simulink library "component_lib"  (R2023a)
settings: Solver=VariableStepAuto  StartTime=0.0  StopTime=10.0  RelTol=1e-3
undefined symbols (not defined in the file or in its folder): component_lib, ECCV_r, KoblenzTrier, mm, par, param_TD04, R1234yf_ph, SigIdentifier, Systems, TH0023_WP120, Thermal, V_nom
libraries: base_lib x166, $bdroot x164, simulink x2, slpidlib x1
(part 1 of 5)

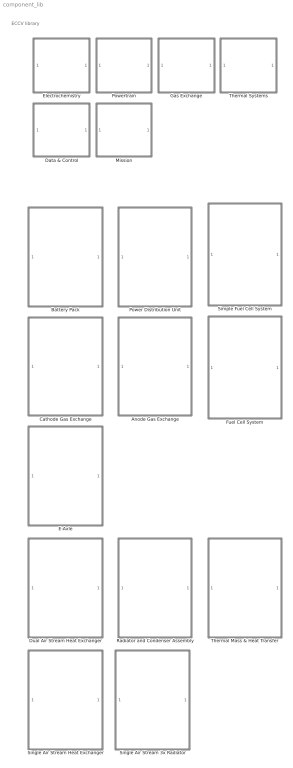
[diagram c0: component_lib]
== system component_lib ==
  note: ECCV library
  Anode Gas Exchange : Subsystem
  Battery Pack : Subsystem  mask{SOC_0=0.5, Nx=74, Ny=6*16}
      mask prompts: SOC_0 "Initial charge [-]:"; Nx "Cells in parallel  [-]:"; Ny "Cells in series [-]:"
      mask init:
      | % parameter struct
      | par = struct;
      | 
      | % Get user-defined parameters
      | par.Ny = eval(get_param(gcb, 'Ny'));
      | par.Nx = eval(get_param(gcb, 'Nx'));
  Cathode Gas Exchange : Subsystem
  Data & Control : Subsystem
  Dual Air Stream Heat Exchanger : Subsystem  mask{HtH=1.1, StS=0.95}
      mask prompts: HtH "Header to header [m]"; StS "Sideplate to sideplate [m]"
  E-Axle : Subsystem  mask{n=3, V_nom=700}
      mask prompts: n "Nr. of motors [-]"; V_nom "Nomnal voltage [V]:"
  Electrochemistry : Subsystem
  Fuel Cell System : Subsystem  mask{n_st=2, n=375}
      mask prompts: n_st "Stacks in series [#]:"; n "Cells per stack [#]:"
  Gas Exchange : Subsystem
  Mission : Subsystem
  Power Distribution Unit : Subsystem  mask{R_bf=1}
      mask prompts: R_bf "Burn-off resistance [Ohm]:"
  Powertrain : Subsystem
  Radiator and Condenser Assembly : Subsystem
  Simple Fuel Cell System : Subsystem  mask{n_st=2, n=375}
      mask prompts: n_st "Stacks in series [#]:"; n "Cells per stack [#]:"
  Single Air Stream 3x Radiator : Subsystem  mask{HtH=1.1, StS=0.95}
      mask prompts: HtH "Header to header [m]"; StS "Sideplate to sideplate [m]"
  Single Air Stream Heat Exchanger : Subsystem  mask{HtH=1.1, StS=0.95}
      mask prompts: HtH "Header to header [m]"; StS "Sideplate to sideplate [m]"
  Thermal Mass & Heat Transfer : Subsystem  mask{n=5, d=2e-3, L=50e-2, m=150, cp=420, T_0=273 + 20}
      mask prompts: n "Channels [-]:"; d "Hydraulic diameter [m]:"; L "Length [m]:"; m "Mass [kg]:"; cp "Heat capacity [J/kgK]:"; T_0 "Initial temperature [K]:"
  Thermal Systems : Subsystem

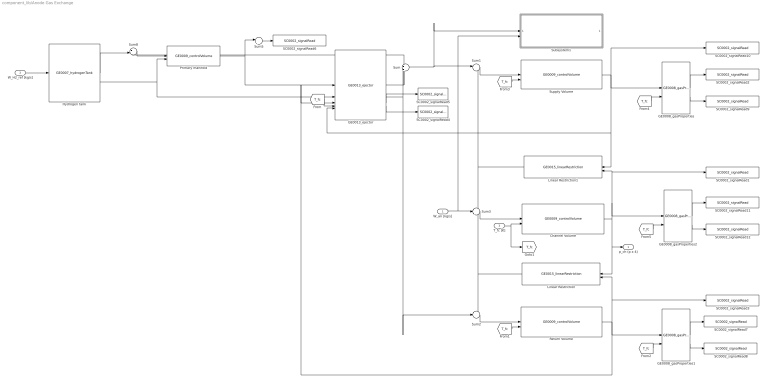
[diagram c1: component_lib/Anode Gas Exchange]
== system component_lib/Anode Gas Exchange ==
  W_an [kg/s] : Inport
  W_H2_ref [kg/s] : Inport  Port=2
  T_fc [K] : Inport  Port=3
  Channel Volume : $bdroot/Gas Exchange/GE0009_controlVolume  V=5e-3  p0=2.5e5  x0_H2=1  x0_O2=0  RH0=0.5
  GE0008_gasProperties : $bdroot/Gas Exchange/GE0008_gasProperties  SystemSampleTime=-1  VariantActivationTime=update diagram  Latency=0  AutoFrameSizeCalculation=off
  GE0008_gasProperties1 : $bdroot/Gas Exchange/GE0008_gasProperties  SystemSampleTime=-1  VariantActivationTime=update diagram  Latency=0  AutoFrameSizeCalculation=off
  GE0008_gasProperties2 : $bdroot/Gas Exchange/GE0008_gasProperties  SystemSampleTime=-1  VariantActivationTime=update diagram  Latency=0  AutoFrameSizeCalculation=off
  GE0013_ejector : $bdroot/Gas Exchange/GE0013_ejector  C_d=1  D_t=1.84e-3  Pi_lin=0.97  c_0=0.78406  c_1=-0.85801
  Hydrogen tank : $bdroot/Gas Exchange/GE0007_hydrogenTank  V=200e-3  T_tank=300  p_out=1.2e5  init_SOC=0.9  m0=5
  Linear Restriction : $bdroot/Gas Exchange/GE0015_linearRestriction  C_d=1e-5
  Linear Restriction1 : $bdroot/Gas Exchange/GE0015_linearRestriction  C_d=1e-5
  Primary manifold : $bdroot/Gas Exchange/GE0009_controlVolume  V=10e-3  p0=5e5  x0_H2=1  x0_O2=0  RH0=0.5
  Return Volume : $bdroot/Gas Exchange/GE0009_controlVolume  V=20e-3  p0=2.5e5  x0_H2=1  x0_O2=0  RH0=0.5
  SC0002_signalRead1 : $bdroot/Data & Control/SC0002_signalRead  SigName=anodeChannelPartialPressure
  SC0002_signalRead10 : $bdroot/Data & Control/SC0002_signalRead  SigName=anodeSupplyPartialPressure
  SC0002_signalRead11 : $bdroot/Data & Control/SC0002_signalRead  SigName=anodeChannelPressure
  SC0002_signalRead12 : $bdroot/Data & Control/SC0002_signalRead  SigName=anodeChannelHumidity
  SC0002_signalRead2 : $bdroot/Data & Control/SC0002_signalRead  SigName=anodeSupplyPressure
  SC0002_signalRead3 : $bdroot/Data & Control/SC0002_signalRead  SigName=anodeReturnPartialPressure
  SC0002_signalRead4 : $bdroot/Data & Control/SC0002_signalRead  SigName=entrainment
  SC0002_signalRead5 : $bdroot/Data & Control/SC0002_signalRead  SigName=recirculation
  SC0002_signalRead6 : $bdroot/Data & Control/SC0002_signalRead  SigName=anodePrimaryPressure
  SC0002_signalRead7 : $bdroot/Data & Control/SC0002_signalRead  SigName=anodeReturnPressure
  SC0002_signalRead8 : $bdroot/Data & Control/SC0002_signalRead  SigName=anodeReturnHumidity
  SC0002_signalRead9 : $bdroot/Data & Control/SC0002_signalRead  SigName=anodeSupplyHumidity
  Subsystem1 : Subsystem
  Sum : Sum  Inputs=+|+
  Sum1 : Sum  Inputs=|+-
  Sum2 : Sum  Inputs=+--
  Sum3 : Sum  Inputs=++-
  Sum5 : Sum  Inputs=1
  Sum8 : Sum  Inputs=-+|
  Supply Volume : $bdroot/Gas Exchange/GE0009_controlVolume  V=20e-3  p0=3e5  x0_H2=1  x0_O2=0  RH0=0.5
  p_ch (p x 4) : Outport
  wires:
  Sum1/1 -> Supply Volume/1
  GE0013_ejector/1 -> Sum/1, Sum8/1
  T_fc [K]/1 -> [T_fc], Channel Volume/2
  GE0013_ejector/4 -> SC0002_signalRead4/1
  GE0013_ejector/3 -> SC0002_signalRead5/1
  Hydrogen tank/2 -> Primary manifold/2, GE0013_ejector/2
  Sum8/1 -> Primary manifold/1
  Hydrogen tank/1 -> Sum8/2
  W_H2_ref [kg/s]/1 -> Hydrogen tank/1
  Sum5/1 -> SC0002_signalRead6/1
  Primary manifold/1 -> GE0013_ejector/1, Sum5/1
  GE0008_gasProperties/1 -> SC0002_signalRead2/1
  GE0013_ejector/2 -> Sum/2, Sum2/2
  Sum/1 -> Subsystem1/1(W_an), Sum1/1
  GE0008_gasProperties1/2 -> SC0002_signalRead8/1
  GE0008_gasProperties1/1 -> SC0002_signalRead7/1
  Linear Restriction/1 -> Sum3/3, Sum2/1
  Sum2/1 -> Return Volume/1
  Supply Volume/1 -> GE0013_ejector/5, Linear Restriction1/1, SC0002_signalRead10/1, GE0008_gasProperties/1
  Return Volume/1 -> SC0002_signalRead3/1, Linear Restriction/2, GE0013_ejector/3, GE0008_gasProperties1/1
  Sum3/1 -> Channel Volume/1
  Linear Restriction1/1 -> Sum1/2, Sum3/1
  W_an [kg/s]/1 -> Subsystem1/2(W_an_reacted), Sum3/2
  [T_fc] -> GE0013_ejector/4
  [T_fc] -> Return Volume/2
  [T_fc] -> GE0008_gasProperties1/2
  [T_fc] -> Supply Volume/2
  [T_fc] -> GE0008_gasProperties/2
  GE0008_gasProperties2/2 -> SC0002_signalRead12/1
  [T_fc] -> GE0008_gasProperties2/2
  Channel Volume/1 -> Linear Restriction/1, p_ch (p x 4)/1, GE0008_gasProperties2/1, SC0002_signalRead1/1, Linear Restriction1/2
  GE0008_gasProperties/2 -> SC0002_signalRead9/1
  GE0008_gasProperties2/1 -> SC0002_signalRead11/1

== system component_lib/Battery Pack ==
  I [A] : Inport
  T [K] : Inport  Port=2
  Battery current : $bdroot/Data & Control/SC0002_signalRead  SigName=batteryCurrent
  Cell current : $bdroot/Data & Control/SC0002_signalRead  SigName=batteryCellCurrent
  Cell voltage : $bdroot/Data & Control/SC0002_signalRead  SigName=batteryCellVoltage
  Constant1 : Constant  Value=Nx
  Constant2 : Constant  Value=Ny
  Constant4 : Constant  Value=Ny
  Constant5 : Constant  Value=Nx
  Divide : Product  Inputs=*/
  EL0001_panasonicNCR18650PF : $bdroot/Electrochemistry/EL0001_panasonicNCR18650PF  init_SOC=SOC_0
  Module voltage : $bdroot/Data & Control/SC0002_signalRead  SigName=batteryVoltage
  Module voltage1 : $bdroot/Data & Control/SC0002_signalRead  SigName=batteryPower
  Product1 : Product
  Product2 : Product  Inputs=3
  Product3 : Product
  SOC : $bdroot/Data & Control/SC0002_signalRead  SigName=stateOfCharge
  V [V] : Outport
  SOC [-] : Outport  Port=2
  Q_gen [J/s] : Outport  Port=3
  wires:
  Product1/1 -> Product3/2, Module voltage/1, V [V]/1
  EL0001_panasonicNCR18650PF/2 -> SOC/1, SOC [-]/1
  Constant2/1 -> Product1/1
  EL0001_panasonicNCR18650PF/1 -> Cell voltage/1, Product1/2
  Divide/1 -> EL0001_panasonicNCR18650PF/1, Cell current/1
  I [A]/1 -> Product3/1, Battery current/1, Divide/1
  Constant1/1 -> Divide/2
  T [K]/1 -> EL0001_panasonicNCR18650PF/2
  EL0001_panasonicNCR18650PF/3 -> Product2/1
  Constant5/1 -> Product2/3
  Constant4/1 -> Product2/2
  Product2/1 -> Q_gen [J/s]/1
  Product3/1 -> Module voltage1/1

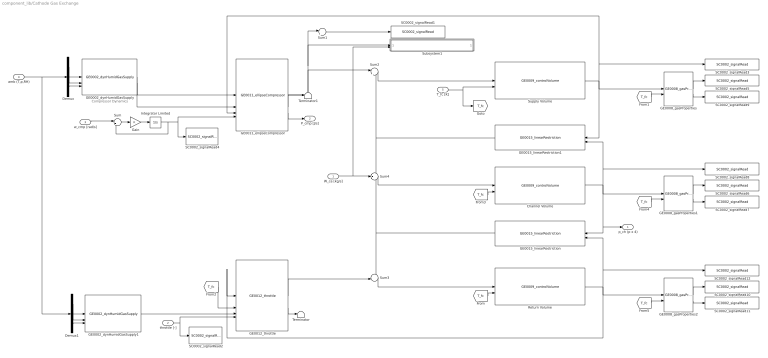
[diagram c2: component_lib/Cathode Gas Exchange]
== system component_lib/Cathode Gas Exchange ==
  note: Compressor Dynamics
  W_ca [kg/s] : Inport
  throttle [-] : Inport  Port=2
  w_cmp [rad/s] : Inport  Port=3
  amb (T,p,RH) : Inport  Port=4
  T_fc [K] : Inport  Port=5
  Channel Volume : $bdroot/Gas Exchange/GE0009_controlVolume  V=10e-3  p0=2.3e5  x0_H2=0  x0_O2=0.21  RH0=0.8
  Demux : Demux  Outputs=3
  Demux1 : Demux  Outputs=3
  GE0002_dynHumidGasSupply : $bdroot/Gas Exchange/GE0002_dynHumidGasSupply  x_H2_dry=0  x_O2_dry=0.21
  GE0002_dynHumidGasSupply1 : $bdroot/Gas Exchange/GE0002_dynHumidGasSupply  x_H2_dry=0  x_O2_dry=0.21
  GE0008_gasProperties : $bdroot/Gas Exchange/GE0008_gasProperties  SystemSampleTime=-1  VariantActivationTime=update diagram  Latency=0  AutoFrameSizeCalculation=off
  GE0008_gasProperties1 : $bdroot/Gas Exchange/GE0008_gasProperties  SystemSampleTime=-1  VariantActivationTime=update diagram  Latency=0  AutoFrameSizeCalculation=off
  GE0008_gasProperties2 : $bdroot/Gas Exchange/GE0008_gasProperties  SystemSampleTime=-1  VariantActivationTime=update diagram  Latency=0  AutoFrameSizeCalculation=off
  GE0011_ellipseCompressor : $bdroot/Gas Exchange/GE0011_ellipseCompressor  w0=15e3
  GE0012_throttle : $bdroot/Gas Exchange/GE0012_throttle  a0=1.3229e-05  a1=9.4736e-05  a2=0.0029  Pi_lin=0.97
  GE0015_linearRestriction : $bdroot/Gas Exchange/GE0015_linearRestriction  C_d=1e-5
  GE0015_linearRestriction1 : $bdroot/Gas Exchange/GE0015_linearRestriction  C_d=1e-5
  Gain : Gain
  Integrator Limited : Integrator  InitialCondition=1e4  LimitOutput=on  UpperSaturationLimit=2e4  LowerSaturationLimit=3e3
  Return Volume : $bdroot/Gas Exchange/GE0009_controlVolume  V=40e-3  p0=2e5  x0_H2=0  x0_O2=0.21  RH0=0.8
  SC0002_signalRead1 : $bdroot/Data & Control/SC0002_signalRead  SigName=compressorFlow
  SC0002_signalRead10 : $bdroot/Data & Control/SC0002_signalRead  SigName=cathodeReturnPressure
  SC0002_signalRead11 : $bdroot/Data & Control/SC0002_signalRead  SigName=cathodeReturnHumidity
  SC0002_signalRead12 : $bdroot/Data & Control/SC0002_signalRead  SigName=cathodeReturnPartialPressure
  SC0002_signalRead2 : $bdroot/Data & Control/SC0002_signalRead  SigName=throttlePosition
  SC0002_signalRead3 : $bdroot/Data & Control/SC0002_signalRead  SigName=cathodeSupplyPartialPressure
  SC0002_signalRead4 : $bdroot/Data & Control/SC0002_signalRead  SigName=compressorSpeed
  SC0002_signalRead5 : $bdroot/Data & Control/SC0002_signalRead  SigName=cathodeSupplyPressure
  SC0002_signalRead6 : $bdroot/Data & Control/SC0002_signalRead  SigName=cathodeChannelPressure
  SC0002_signalRead7 : $bdroot/Data & Control/SC0002_signalRead  SigName=cathodeChannelHumidity
  SC0002_signalRead8 : $bdroot/Data & Control/SC0002_signalRead  SigName=cathodeChannelPartialPressure
  SC0002_signalRead9 : $bdroot/Data & Control/SC0002_signalRead  SigName=cathodeSupplyHumidity
  Subsystem1 : Subsystem
  Sum : Sum  Inputs=|+-
  Sum1 : Sum  Inputs=1
  Sum2 : Sum  Inputs=|+-
  Sum3 : Sum  Inputs=+-|
  Sum4 : Sum  Inputs=++-
  Supply Volume : $bdroot/Gas Exchange/GE0009_controlVolume  V=40e-3  p0=2.5e5  x0_H2=0  x0_O2=0.21  RH0=0.8
  Terminator : Terminator
  Terminator1 : Terminator
  p_ch (p x 4) : Outport
  P_cmp [J/s] : Outport  Port=2
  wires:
  Sum1/1 -> SC0002_signalRead1/1
  Gain/1 -> Integrator Limited/1
  Integrator Limited/1 -> SC0002_signalRead4/1, GE0011_ellipseCompressor/4, Sum/2
  Sum/1 -> Gain/1
  w_cmp [rad/s]/1 -> Sum/1
  GE0002_dynHumidGasSupply/1 -> GE0011_ellipseCompressor/1
  GE0002_dynHumidGasSupply1/1 -> GE0012_throttle/3
  GE0002_dynHumidGasSupply/2 -> GE0011_ellipseCompressor/2
  GE0011_ellipseCompressor/1 -> Sum2/1, Sum1/1, Subsystem1/1(W_ca)
  throttle [-]/1 -> SC0002_signalRead2/1, GE0012_throttle/4
  Demux/1 -> GE0002_dynHumidGasSupply/1
  Demux/2 -> GE0002_dynHumidGasSupply/2
  Demux/3 -> GE0002_dynHumidGasSupply/3
  Demux1/1 -> GE0002_dynHumidGasSupply1/1
  Demux1/2 -> GE0002_dynHumidGasSupply1/2
  Demux1/3 -> GE0002_dynHumidGasSupply1/3
  amb (T,p,RH)/1 -> Demux/1, Demux1/1
  GE0008_gasProperties/1 -> SC0002_signalRead5/1
  Supply Volume/1 -> GE0015_linearRestriction1/1, GE0008_gasProperties/1, GE0011_ellipseCompressor/3, SC0002_signalRead3/1
  GE0008_gasProperties/2 -> SC0002_signalRead9/1
  Sum2/1 -> Supply Volume/1
  GE0011_ellipseCompressor/3 -> P_cmp [J/s]/1
  GE0015_linearRestriction/1 -> Sum4/3, Sum3/1
  T_fc [K]/1 -> [T_fc], Supply Volume/2
  Sum3/1 -> Return Volume/1
  GE0012_throttle/1 -> Sum3/2
  GE0012_throttle/2 -> Terminator/1
  GE0011_ellipseCompressor/2 -> Terminator1/1
  [T_fc] -> Return Volume/2
  [T_fc] -> GE0008_gasProperties/2
  [T_fc] -> GE0012_throttle/2
  Channel Volume/1 -> p_ch (p x 4)/1, GE0015_linearRestriction/1, GE0008_gasProperties1/1, GE0015_linearRestriction1/2, SC0002_signalRead8/1
  W_ca [kg/s]/1 -> Sum4/2, Subsystem1/2(W_ca_reacted)
  GE0015_linearRestriction1/1 -> Sum4/1, Sum2/2
  Sum4/1 -> Channel Volume/1
  [T_fc] -> Channel Volume/2
  [T_fc] -> GE0008_gasProperties1/2
  GE0008_gasProperties1/1 -> SC0002_signalRead6/1
  GE0008_gasProperties1/2 -> SC0002_signalRead7/1
  GE0008_gasProperties2/1 -> SC0002_signalRead10/1
  GE0008_gasProperties2/2 -> SC0002_signalRead11/1
  [T_fc] -> GE0008_gasProperties2/2
  Return Volume/1 -> GE0008_gasProperties2/1, GE0012_throttle/1, GE0015_linearRestriction/2, SC0002_signalRead12/1

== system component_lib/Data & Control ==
  DC0007_cathodeFlowControl : Subsystem  mask{lambda_O2_ref=2, n_cell=455}
      mask prompts: lambda_O2_ref "Oxygen stoich. reference [-]:"; n_cell "Nr. of cells [-]:"
  SC0002_signalRead : Subsystem  mask{SigName=SigIdentifier}
      mask prompts: SigName "Signal identifier:"
      mask init:
      | % set name of input port
      | blockNames = Simulink.findBlocks(gcb);
      | set(blockNames(1), 'Name', SigName);
      | 
      | % log input port
      | ph = get_param([gcb, '/', SigName], 'PortHandles');
      | set_param(ph.Outport(1), 'DataLogging', 'on')
      | 
      | % set signal name in goto tag
      | set_param([gcb, '/', 'Goto'], 'GotoTag', SigName)
  SC0003_signalWrite : Subsystem  mask{SigName=SigIdentifier}
      mask prompts: SigName "Signal identifier:"
      mask init:
      | % set signal name in goto tag
      | set_param([gcb, '/', 'From'], 'GotoTag', SigName)

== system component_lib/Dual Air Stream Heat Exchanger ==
  AMB: (T,p,RH) : Inport
  v [m/s] : Inport  Port=2
  Q_cds [J/s] : Inport  Port=3
  rel_fan_speed [-] : Inport  Port=4
  CL: (T1,p1,W1) : Inport  Port=5
  Demux : Demux  Outputs=3
  Mux : Mux  Inputs=3
  Radiator core - behind CDS : $bdroot/Thermal Systems/TH0002_radiatorCore  HtH=0.35  StS=0.95  radmodel=52 mm
  Radiator core - exposed : $bdroot/Thermal Systems/TH0002_radiatorCore  HtH=1.1-0.35  StS=0.95  radmodel=52 mm
  TH0003_coolantTank : $bdroot/Thermal Systems/TH0003_coolantTank  StS=0.95  D_con=0.055  T_0=286  radmodel=52 mm
  TH0003_coolantTank1 : $bdroot/Thermal Systems/TH0003_coolantTank  StS=0.95  D_con=0.055  T_0=286  radmodel=52 mm
  TH0004_radiatorPlugFlow : $bdroot/Thermal Systems/TH0004_radiatorPlugFlow  HtH=1.1  StS=0.95  T_0=286  radmodel=52 mm
  TH0005_flowSplit : $bdroot/Thermal Systems/TH0005_flowSplit  SystemSampleTime=-1  VariantActivationTime=update diagram  Latency=0  AutoFrameSizeCalculation=off
  TH0006_flowConfluence : $bdroot/Thermal Systems/TH0006_flowConfluence  gain=0.01
  TH0007_airRestriction : $bdroot/Thermal Systems/TH0007_airRestriction  A=0.8  zeta=0.3
  TH0007_airRestriction1 : $bdroot/Thermal Systems/TH0007_airRestriction  A=1  zeta=2.5
  TH0008_condenser : $bdroot/Thermal Systems/TH0008_condenser  HtH=0.85  StS=0.35  cdsmodel=18.8 mm
  TH0009_intake : $bdroot/Thermal Systems/TH0009_intake  zeta=0.9
  TH0010_fan : $bdroot/Thermal Systems/TH0010_fan  n_fan=4
  TH0011_outletFlowBalance : $bdroot/Thermal Systems/TH0011_outletFlowBalance  gain=0.05
  P_fan [J/s] : Outport
  CL: (T2,p2,W2) : Outport  Port=2
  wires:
  Demux/2 -> Mux/2, [p_amb]
  Demux/1 -> Mux/1
  AMB: (T,p,RH)/1 -> Demux/1
  TH0003_coolantTank1/1 -> CL: (T2,p2,W2)/1
  TH0010_fan/2 -> P_fan [J/s]/1
  rel_fan_speed [-]/1 -> TH0010_fan/2
  TH0005_flowSplit/1 -> TH0008_condenser/1
  v [m/s]/1 -> TH0009_intake/2
  TH0007_airRestriction/1 -> TH0005_flowSplit/1
  TH0004_radiatorPlugFlow/1 -> TH0003_coolantTank1/1
  TH0007_airRestriction1/1 -> TH0011_outletFlowBalance/1
  TH0003_coolantTank/1 -> Radiator core - behind CDS/2
  Q_cds [J/s]/1 -> TH0008_condenser/2
  CL: (T1,p1,W1)/1 -> TH0003_coolantTank/1
  TH0006_flowConfluence/2 -> TH0005_flowSplit/2
  TH0006_flowConfluence/1 -> TH0010_fan/1
  Mux/1 -> TH0009_intake/1
  TH0005_flowSplit/2 -> [air_22]
  TH0009_intake/1 -> TH0007_airRestriction/1
  TH0008_condenser/1 -> Radiator core - behind CDS/1
  Radiator core - behind CDS/2 -> TH0006_flowConfluence/1
  Radiator core - exposed/2 -> TH0006_flowConfluence/2
  Radiator core - behind CDS/3 -> Radiator core - exposed/2
  [p_amb] -> TH0011_outletFlowBalance/2
  [air_22] -> Radiator core - exposed/1
  TH0010_fan/1 -> TH0007_airRestriction1/1
  Radiator core - exposed/3 -> TH0004_radiatorPlugFlow/1
  TH0011_outletFlowBalance/1 -> [W_in]
  [W_in] -> Mux/3

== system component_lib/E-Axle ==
  note: Input as % of max. torque at current speed
  Tq_sig [-] : Inport
  gear [-] : Inport  Port=2
  V [V] : Inport  Port=3
  w_w [rad/s] : Inport  Port=4
  Constant1 : Constant  Value=V_nom
  Constant3 : Constant
  Current sensor : $bdroot/Data & Control/SC0002_signalRead  SigName=motorCurrent
  Divide : Product  Inputs=**/
  Divide1 : Product  Inputs=**
  Gain : Gain  Gain=n
  Gain1 : Gain  Gain=n
  Gain2 : Gain  Gain=n
  Gain3 : Gain  Gain=-1
  Max torque : $bdroot/Data & Control/SC0002_signalRead  SigName=maxMotorTorque
  Min torque : $bdroot/Data & Control/SC0002_signalRead  SigName=minMotorTorque
  PT0002_simpleMotor : $bdroot/Powertrain/PT0002_simpleMotor  T_s=0.1
  PT0003_gearBox : $bdroot/Powertrain/PT0003_gearBox  fd_ratio=2  gear_ratios=[5 3.8 2.3 1.15]  eta_gb=0.98
  Saturation2 : Saturate  UpperLimit=1  LowerLimit=-1
  Saturation3 : Saturate  UpperLimit=476  LowerLimit=0
  Saturation4 : Saturate  UpperLimit=V_nom  LowerLimit=0
  Speed sensor : $bdroot/Data & Control/SC0002_signalRead  SigName=motorSpeed
  Torque sensor : $bdroot/Data & Control/SC0002_signalRead  SigName=motorTorque
  speed-Torque map1 : Lookup_n-D  NumberOfTableDimensions=1  BreakpointsForDimension1=|  Table=|  ExtrapMethod=Clip  UseLastTableValue=on  InternalRulePriority=Speed  RndMeth=Simplest
      | [25.2590673575129
      | 34.9740932642487
      | 43.3937823834197
      | 51.1658031088083
      | 55.6994818652850
      | 64.1191709844560
      | 65.4145077720207
      | 67.3575129533679
      | 68.0051813471503
      | 69.9481865284974
      | 71.2435233160622
      | 73.1865284974093
      | 75.7772020725389
      | 76.4248704663213
      | 78.3678756476684
      | 81.6062176165803
      | 82.9015544041451
      | 86.1398963730570
      | 88.0829015544041
      | 90.0259067357513
      | 94.5595854922280
      | 97.1502590673575
      | 100.388601036269
      | 103.6269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
      | [1991.26637554585
      | 1997.08879184862
      | 1994.17758369723
      | 1994.17758369723
      | 1994.17758369723
      | 1991.26637554585
      | 1944.68704512373
      | 1921.39737991266
      | 1854.43959243086
      | 1816.59388646288
      | 1787.48180494905
      | 1700.14556040757
      | 1671.03347889374
      | 1621.54294032023
      | 1548.76273653566
      | 1513.82823871907
      | 1438.13682678311
      | 1391.55749636099
      | 1339.15574963610
      | 1280.93158660844
      | 1225.61863173217
      | 1176.12809315866
      | 1129.54876273654
      | 1085.880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
  Tq_axle [Nm] : Outport
  I_em [A] : Outport  Port=2
  Q_gen [J/s] : Outport  Port=3
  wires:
  Gain2/1 -> Tq_axle [Nm]/1
  PT0003_gearBox/1 -> Gain2/1
  PT0002_simpleMotor/3 -> Gain/1
  Gain1/1 -> Current sensor/1, I_em [A]/1
  PT0002_simpleMotor/1 -> PT0003_gearBox/1, Torque sensor/1
  Constant3/1 -> PT0003_gearBox/4
  gear [-]/1 -> PT0003_gearBox/3
  PT0003_gearBox/2 -> Divide/1, PT0002_simpleMotor/3, Speed sensor/1
  w_w [rad/s]/1 -> PT0003_gearBox/2
  PT0002_simpleMotor/2 -> Gain1/1
  Gain/1 -> Q_gen [J/s]/1
  Gain3/1 -> Min torque/1
  V [V]/1 -> PT0002_simpleMotor/2, Saturation4/1
  speed-Torque map1/1 -> Divide1/2, Gain3/1, Max torque/1
  Saturation2/1 -> Divide1/1
  Saturation4/1 -> Divide/3
  Saturation3/1 -> speed-Torque map1/1
  Divide1/1 -> PT0002_simpleMotor/1
  Tq_sig [-]/1 -> Saturation2/1
  Constant1/1 -> Divide/2
  Divide/1 -> Saturation3/1

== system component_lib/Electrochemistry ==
  EL0001_panasonicNCR18650PF : Subsystem  mask{init_SOC=0.2380}
      mask prompts: init_SOC "Initial SOC [-]:"
      mask init:
      | % parameter struct
      | par = struct;
      | 
      | % Get user-defined parameters
      | par.init_SOC   = init_SOC;
  EL0004_buckCCM : Subsystem  mask{R=1e-3, C=1, L=1e-6, V_init=400}
      mask prompts: R "Resistance [Ohm]:"; C "Capacity [F]:"; L "Inductance [H]:"; V_init "Voltage initial condition [V]:"
  EL0005_boostCCM : Subsystem  mask{C=1, L=1, eta=0.9, V_init=420}
      mask prompts: C "Capacity [F]:"; L "Inductance [H]:"; eta "Efficiency [-]:"; V_init "Voltage initial condition [V]:"
  EL0006_busDC : Subsystem  mask{R=1e-3, C=1, L=912e-9, V_init=420}
      mask prompts: R "Resistance [Ohm]:"; C "Capacitance [F]:"; L "Inductance [H]:"; V_init "Voltage initial condition [V]:"
  EL0007_pukrushpan2004 : Subsystem  mask{U_0=1, j_0=1e-3, alpha=0.25, ASR=1e-1, A_fc=300}
      mask prompts: U_0 "Open circuit voltage [V]:"; j_0 "Exchange current density [A/cm2]:"; alpha "Act. bar. symmetry [-]:"; ASR "Area specific resistance [ohm*cm2]:"; A_fc "Membrane area [cm2]:"
      mask init:
      | % parameter struct
      | par = struct;
      | 
      | % Get user-defined parameters
      | par.j_0   = j_0;
      | par.alpha = alpha;
      | par.ASR   = ASR;
      | par.U_0   = U_0;
      | par.A_fc  = A_fc;
      | 
      | % membrane thickness
      | par.t_m    = 0.01275;
      | 
      | % Molar mass - [kg/mol]
      | par.M_j  = [0.002;
      |             0.032;
      |             0.018;
      |             0.028];    
      | 
      | % Specific heat - [J/kg*K]        
      | par.cp_j = [14.43e3;
      |             0.928e3;
      |             1.996e3;
      |             1.041e3];  
      | 
      | % Universal gas constant - [J/(mol*K)]   
      | par.R  = 8.314;         
      | 
      | % Specific gas constant [J/kg*K]
      | par.R_j = par.R ./ par.M_j;
  EL0008_dcdcConverter : Subsystem  mask{eta_up=0.99, eta_down=0.99}
      mask prompts: eta_up "Efficiency up [-]"; eta_down "Efficiency down [-]"
      mask init:
      | par = struct;
      | par.eta_up = eta_up;
      | par.eta_down = eta_down;
  EL0010_superCapacitor : Subsystem  mask{C=1, V_bus0=700}
      mask prompts: C "Capacity [F]:"; V_bus0 "Initial voltage [V]:"

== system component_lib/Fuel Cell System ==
  I [A] : Inport
  throttle [-] : Inport  Port=2
  w_cmp [rad/s] : Inport  Port=3
  W_H2_ref [kg/s] : Inport  Port=4
  amb (T,p,RH) : Inport  Port=5
  T [K] : Inport  Port=6
  Anode Gas Exchange : $bdroot/Anode Gas Exchange  SystemSampleTime=-1  VariantActivationTime=update diagram  Latency=0  AutoFrameSizeCalculation=off
  Cathode Gas Exchange : $bdroot/Cathode Gas Exchange  SystemSampleTime=-1  VariantActivationTime=update diagram  Latency=0  AutoFrameSizeCalculation=off
  Constant4 : Constant  Value=n
  EL0007_pukrushpan2004 : $bdroot/Electrochemistry/EL0007_pukrushpan2004  U_0=1  j_0=1e-3  alpha=0.25  ASR=1e-1  A_fc=420
  F0010_vaporSaturationPressure.m : base_lib/F0010_gasFlow/F0010_vaporSaturationPressure.m  SystemSampleTime=-1  VariantActivationTime=update diagram  Latency=0  AutoFrameSizeCalculation=off
  Gain{,1..3} (4 alike) : Gain  Gain=n_st
  Gain4 : Gain  Gain=1/420
  Product{1..5} (5 alike) : Product
  SC0002_signalRead1 : $bdroot/Data & Control/SC0002_signalRead  SigName=fuelCellVoltage
  SC0002_signalRead2 : $bdroot/Data & Control/SC0002_signalRead  SigName=fuelCellCurrent
  SC0002_signalRead3 : $bdroot/Data & Control/SC0002_signalRead  SigName=membraneWaterContent
  SC0002_signalRead4 : $bdroot/Data & Control/SC0002_signalRead  SigName=fuelCellPower
  SC0002_signalRead5 : $bdroot/Data & Control/SC0002_signalRead  SigName=vaporSaturationPressure
  SC0002_signalRead6 : $bdroot/Data & Control/SC0002_signalRead  SigName=singleCellVoltage
  SC0002_signalRead7 : $bdroot/Data & Control/SC0002_signalRead  SigName=compressorPower
  SC0002_signalRead8 : $bdroot/Data & Control/SC0002_signalRead  SigName=currentDensity
  Subsystem1 : Subsystem
  V [V] : Outport
  Q_gen [J/s] : Outport  Port=2
  P_cmp [J/s] : Outport  Port=3
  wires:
  Product1/1 -> Gain1/1
  EL0007_pukrushpan2004/1 -> Product1/1, SC0002_signalRead6/1
  Product2/1 -> [W_an], Gain/1
  Product5/1 -> [W_ca]
  Constant4/1 -> Product1/2, Product2/2, Product5/2, Product3/2
  I [A]/1 -> EL0007_pukrushpan2004/1, SC0002_signalRead2/1, Product4/1, Gain4/1
  EL0007_pukrushpan2004/3 -> Product5/1
  EL0007_pukrushpan2004/2 -> Product2/1
  EL0007_pukrushpan2004/5 -> Product3/1
  Product4/1 -> SC0002_signalRead4/1
  EL0007_pukrushpan2004/4 -> SC0002_signalRead3/1
  T [K]/1 -> F0010_vaporSaturationPressure.m/1, Anode Gas Exchange/3, Cathode Gas Exchange/5, EL0007_pukrushpan2004/4, EL0007_pukrushpan2004/5, EL0007_pukrushpan2004/6
  Cathode Gas Exchange/2 -> Gain3/1
  amb (T,p,RH)/1 -> Cathode Gas Exchange/4
  F0010_vaporSaturationPressure.m/1 -> SC0002_signalRead5/1
  Cathode Gas Exchange/1 -> EL0007_pukrushpan2004/3
  [W_ca] -> Cathode Gas Exchange/1
  Gain3/1 -> SC0002_signalRead7/1, P_cmp [J/s]/1
  Gain/1 -> Subsystem1/1(In1)
  Gain1/1 -> V [V]/1, SC0002_signalRead1/1, Product4/2
  Product3/1 -> Gain2/1
  Gain2/1 -> Q_gen [J/s]/1
  throttle [-]/1 -> Cathode Gas Exchange/2
  w_cmp [rad/s]/1 -> Cathode Gas Exchange/3
  Anode Gas Exchange/1 -> EL0007_pukrushpan2004/2
  [W_an] -> Anode Gas Exchange/1
  Gain4/1 -> SC0002_signalRead8/1
  W_H2_ref [kg/s]/1 -> Anode Gas Exchange/2

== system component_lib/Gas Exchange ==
  GE0001_humidGasSupply : Subsystem  mask{p_tot=1.01e5, x_H2=0, x_O2=0.21, RH=0, T=300}
      mask prompts: p_tot "Pressure [Pa]:"; x_H2 "Mole fraction dry H2 [-]:"; x_O2 "Mole fraction dry O2 [-]:"; RH "Relative humidity [-]:"; T "Temperature [K]:"
      mask init:
      | % parameter struct
      | par = struct;
      | 
      | par.p_tot = p_tot;
      | par.x_H2  = x_H2;
      | par.x_O2  = x_O2;
      | par.RH    = RH;
      | par.T     = T;
      | 
      | % par.p_tot = eval(get_param(gcb, 'p_tot'));
      | % par.x_H2  = eval(get_param(gcb, 'x_H2'));
      | % par.x_O2  = eval(get_param(gcb, 'x_O2'));
      | % par.RH    = eval(get_param(gcb, 'RH'));
      | % par.T     = eval(get_param(gcb, 'T'));
      | 
      | 
      | 
      | % Fixed parameters
      | par.R     = 8.314;  % [J/(mol*K)] - universal gas constant
      | par.M_N2  = 0.028;  % [kg/mol] - nitrogen molecular weight
      | par.M_H2O = 0.018;  % [kg/mol] - water
  GE0002_dynHumidGasSupply : Subsystem  mask{x_H2_dry=0, x_O2_dry=0.21}
      mask prompts: x_H2_dry "Mole-fraction dry hydrogen [-]:"; x_O2_dry "Mole-fraction dry oxygen [-]:"
      mask init:
      | % parameter struct
      | par = struct;
      | 
      | % Fixed parameters
      | par.R     = 8.314; % [J/(mol*K)] - universal gas constant
      | par.M_N2  = 0.028; % [kg/mol] - nitrogen molecular weight
      | par.M_H2O = 0.018; % [kg/mol] - water
  GE0007_hydrogenTank : Subsystem  mask{V=200e-3, T_tank=300, p_out=1.2e5, init_SOC=0.9, m0=5}
      mask prompts: V "Volume [m3]:"; T_tank "Tank temperature [K]:"; p_out "Outlet pressure [Pa]"; init_SOC "Initial charge [-]"; m0 "Total capacity [kg]:"
      mask init:
      | % parameter struct
      | par = struct;
      | 
      | % Get user-specified parameters
      | % par.V        = eval(get_param(gcb, 'V'));
      | % par.T_tank   = eval(get_param(gcb, 'T_tank'));
      | % par.p_out    = eval(get_param(gcb, 'p_out'));
      | % par.init_SOC = eval(get_param(gcb, 'init_SOC'));
      | % par.m0       = eval(get_param(gcb, 'm0'));
      | 
      | par.V        = V;
      | par.T_tank   = T_tank;
      | par.p_out    = p_out;
      | par.init_SOC = init_SOC;
      | par.m0       = m0;
      | 
      | 
      | % Standard state values
      | par.T0 = 298.15;  % [K]     - standard state temperature
      | par.h0 = 7.9260e3; % [J/mol] - standard state enthalpy
      | 
      | % Molar mass - [kg/mol]
      | par.M_j  = [0.002;
      |             0.032;
      |             0.018;
      |             0.028];    
      | 
      | % Specific heat - [J/kg*K]        
      | par.cp_j = [14.43e3;
      |             0.928e3;
      |             1.996e3;
      |             1.041e3];  
      | 
      | % Universal gas constant - [J/(mol*K)]   
      | par.R  = 8.314;         
      | 
      | % Specific gas constant [J/kg*K]
      | par.R_j = par.R ./ par.M_j;
  GE0008_gasProperties : Subsystem
  GE0009_controlVolume : Subsystem  mask{V=1.5833e-05, p0=1.01e5, x0_H2=0, x0_O2=0.21, RH0=0}
      mask prompts: V "Volume [m3]:"; p0 "Pressure [Pa]:"; x0_H2 "Mole fraction dry H2 [-]:"; x0_O2 "Mole fraction dry O2 [-]:"; RH0 "Relative humidity [-]:"
      mask init:
      | % parameter struct
      | par = struct;
      | 
      | % Get user-specified parameters
      | % par.V   = eval(get_param(gcb, 'V'));
      | par.V = V;
      | 
      | % initial conditions
      | par.p0    = p0;
      | par.x0_H2 = x0_H2;
      | par.x0_O2 = x0_O2;
      | par.RH0   = RH0;
      | 
      | % Molar mass - [kg/mol]
      | par.M_j  = [0.002;
      |             0.032;
      |             0.018;
      |             0.028];    
      | 
      | % Specific heat - [J/kg*K]        
      | par.cp_j = [14.43e3;
      |             0.928e3;
      |             1.996e3;
      |             1.041e3];  
      | 
      | % Universal gas constant - [J/(mol*K)]   
      | par.R  = 8.314;         
      | 
      | % Specific gas constant [J/kg*K]
      | par.R_j = par.R ./ par.M_j;
  GE0010_compressibleRestriction : Subsystem  mask{C_d=1, D_t=1.84e-3, Pi_lin=0.97}
      mask prompts: C_d "Discharge coefficient [-]:"; D_t "Throat diameter [m]:"; Pi_lin "Lin. region  [-]"
      mask init:
      | % Check side
      | par = struct;
      | 
      | % parameters
      | par.C_d     = C_d;
      | par.Pi_lin  = Pi_lin;
      | par.D_t     = D_t;
      | 
      | % Molar mass - [kg/mol]
      | par.M_j  = [0.002;
      |             0.032;
      |             0.018;
      |             0.028];    
      | 
      | % Specific heat - [J/kg*K]        
      | par.cp_j = [14.43e3;
      |             0.928e3;
      |             1.996e3;
      |             1.041e3];  
      | 
      | % Universal gas constant - [J/(mol*K)]   
      | par.R  = 8.314;         
      | 
      | % Specific gas constant [J/kg*K]
      | par.R_j = par.R ./ par.M_j;
  GE0011_ellipseCompressor : Subsystem  mask{compressor_parameters=param_TD04.mat, w0=3e3}
      mask prompts: compressor_parameters "Parameter set:"; w0 "Initial speed [rad/s]:"
      mask init:
      | % parameter struct
      | % par = struct;
      | 
      | 
      | 
      | % find compressor models
      | compressorMaps = dir(fullfile('models/F0011_ellipseCompressor','*.mat'));
      | compressorMaps = {compressorMaps.name};
      | 
      | % update popup_list
      | msk = Simulink.Mask.get(gcb);
      | msk.Parameters(1).TypeOptions = compressorMaps;
      | 
      | % set profile
      | % try
      |     load(msk.Parameters(1).Value);
      | % end
      | 
      | % Get user-specified parameters
      | % par.w0   = eval(get_param(gcb, 'w0'));
      | par.w0   = w0;
      | 
      | 
      | % % Compressor parameters
      | % par.C_Wch       = [0.791459084209095;0.278369840595707;2.56393896117876;1.42688664691882];
      | % par.C_PIch      = [0.0903657853262553;0.467638667413134;4.35616456423884]; 
      | % par.C_Wzs       = [0.851951915665070;2.98625689994966];
      | % par.C_PIzs      = [1.24697676678299;2.08506798865712];
      | % par.C_cur       = [2.08068646432419;4.30416619749832;5.84893356036723];
      | % par.Gamma_PIcs  = [0.500000000000000];
      | % par.C_s         = [1.47023010236244];
      | % par.C_b         = [1.806586538255675;-0.642454577867690];
      | % par.C_a         = [0.863755184943499;0.033339263835893;24.999999984802365];
      | % par.C_loss      = 0.009455201151738;
      | % par.T_ref       =  298;
      | % par.p_ref       = 100000;
      | % par.Nc_max_map  = 1.860592187500000e+05;
      | % par.Wc_max_map  = 0.252151000000000;
      | % par.PI_max_map  = 2.766539113153419;
      | % par.Delta_h_max = 1.738661132271557e+05;
      | % par.gamma_air   = 1.397693997445722;
      | % par.rho1        = 1.169072149521521;
      | % par.D_2         = 0.056300000000000;
      | % par.Cp_air      = 1.008800956523303e+03;
      | % par.alpha_kPiW0 = 1.645763320284325;
      | % par.J_c         = 1.730000000000000e-05;
      | % par.c_fric      = 1e-6;
      | 
      | 
      | % Molar mass - [kg/mol]
      | par.M_j  = [0.002;
      |             0.032;
      |             0.018;
      |             0.028];    
      | 
      | % Specific heat - [J/kg*K]        
      | par.cp_j = [14.43e3;
      |             0.928e3;
      |             1.996e3;
      |             1.041e3];  
      | 
      | % Universal gas constant - [J/(mol*K)]   
      | par.R  = 8.314;         
      | 
      | % Specific gas constant [J/kg*K]
      | par.R_j = par.R ./ par.M_j;
  GE0012_throttle : Subsystem  mask{a0=1.3229e-05, a1=9.4736e-05, a2=0.0029, Pi_lin=0.97}
      mask prompts: Pi_lin "Lin. region  [-]"
      mask init:
      | % Check side
      | par = struct;
      | 
      | % parameters
      | par.Pi_lin  = Pi_lin;
      | 
      | par.C_d = 1;
      | par.a0 = a0;
      | par.a1 = a1;
      | par.a2 = a2;
      | 
      | % Molar mass - [kg/mol]
      | par.M_j  = [0.002;
      |             0.032;
      |             0.018;
      |             0.028];    
      | 
      | % Specific heat - [J/kg*K]        
      | par.cp_j = [14.43e3;
      |             0.928e3;
      |             1.996e3;
      |             1.041e3];  
      | 
      | % Universal gas constant - [J/(mol*K)]   
      | par.R  = 8.314;         
      | 
      | % Specific gas constant [J/kg*K]
      | par.R_j = par.R ./ par.M_j;
  GE0013_ejector : Subsystem  mask{C_d=1, D_t=1.84e-3, Pi_lin=0.97, c_0=0.78406, c_1=-0.85801}
      mask prompts: C_d "Discharge coefficient [-]:"; D_t "Nozzle throat diameter [m]:"; Pi_lin "Linear region [-]:"; c_0 "c0"; c_1 "c1"
      mask init:
      | % parameter struct
      | par = struct;
      | 
      | % Get user-specified parameters
      | % par.C_d    = eval(get_param(gcb, 'C_d'));
      | % par.D_t    = eval(get_param(gcb, 'D_t'));
      | % par.Pi_lin = eval(get_param(gcb, 'Pi_lin'));
      | % par.c_0     = eval(get_param(gcb, 'c_0'));
      | % par.c_1     = eval(get_param(gcb, 'c_1'));
      | 
      | par.C_d    = C_d;
      | par.D_t    = D_t;
      | par.Pi_lin = Pi_lin;
      | par.c_0    = c_0;
      | par.c_1    = c_1;
      |  
      | % Molar mass - [kg/mol]
      | par.M_j  = [0.002;
      |             0.032;
      |             0.018;
      |             0.028];    
      | 
      | % Specific heat - [J/kg*K]        
      | par.cp_j = [14.43e3;
      |             0.928e3;
      |             1.996e3;
      |             1.041e3];  
      | 
      | % Universal gas constant - [J/(mol*K)]   
      | par.R  = 8.314;         
      | 
      | % Specific gas constant [J/kg*K]
      | par.R_j = par.R ./ par.M_j;
  GE0014_flowValve : Subsystem  mask{C_d=1, D_t=1.84e-3, Pi_lin=0.97}
      mask prompts: C_d "Discharge coefficient [-]:"; D_t "Throat diameter [m]:"; Pi_lin "Lin. region  [-]"
      mask init:
      | % Check side
      | par = struct;
      | 
      | % parameters
      | par.C_d     = C_d;
      | par.Pi_lin  = Pi_lin;
      | par.D_t     = D_t;
      | 
      | % Molar mass - [kg/mol]
      | par.M_j  = [0.002;
      |             0.032;
      |             0.018;
      |             0.028];    
      | 
      | % Specific heat - [J/kg*K]        
      | par.cp_j = [14.43e3;
      |             0.928e3;
      |             1.996e3;
      |             1.041e3];  
      | 
      | % Universal gas constant - [J/(mol*K)]   
      | par.R  = 8.314;         
      | 
      | % Specific gas constant [J/kg*K]
      | par.R_j = par.R ./ par.M_j;
  GE0015_linearRestriction : Subsystem  mask{C_d=4.7083e-08}
      mask prompts: C_d "Discharge coefficient [-]:"
      mask init:
      | % Check side
      | par = struct;
      | 
      | % parameters
      | % par.C_d     = eval(get_param(gcb, 'C_d'));
      | % par.tan_par = eval(get_param(gcb, 'tan_par'));
      | 
      | par.C_d     = C_d;
      | 
      | % Molar mass - [kg/mol]
      | par.M_j  = [0.002;
      |             0.032;
      |             0.018;
      |             0.028];    
      | 
      | % Specific heat - [J/kg*K]        
      | par.cp_j = [14.43e3;
      |             0.928e3;
      |             1.996e3;
      |             1.041e3];  
      | 
      | % Universal gas constant - [J/(mol*K)]   
      | par.R  = 8.314;         
      | 
      | % Specific gas constant [J/kg*K]
      | par.R_j = par.R ./ par.M_j;
  GE0016_simpleCompressor : Subsystem  mask{eta=0.7}
      mask prompts: eta "Efficiency [-]:"
  GE0017_humidifier : Subsystem  mask{T_s=30, gain=1}
      mask prompts: T_s "Time constant [s]:"; gain "Gain [RH -> Flow]:"
      mask init:
      | % parameter struct
      | par = struct;
      | 
      | 
      | % Molar mass - [kg/mol]
      | par.M_j  = [0.002;
      |             0.032;
      |             0.018;
      |             0.028];    
      | 
      | % Specific heat - [J/kg*K]        
      | par.cp_j = [14.43e3;
      |             0.928e3;
      |             1.996e3;
      |             1.041e3];  
      | 
      | % Universal gas constant - [J/(mol*K)]   
      | par.R  = 8.314;         
      | 
      | % Specific gas constant [J/kg*K]
      | par.R_j = par.R ./ par.M_j;
  GE0018_condenser : Subsystem  mask{T_s=1, gain=1}
      mask prompts: T_s "Time constant [s]:"; gain "Gain [RH -> Flow]:"
      mask init:
      | % parameter struct
      | par = struct;
      | 
      | 
      | % Molar mass - [kg/mol]
      | par.M_j  = [0.002;
      |             0.032;
      |             0.018;
      |             0.028];    
      | 
      | % Specific heat - [J/kg*K]        
      | par.cp_j = [14.43e3;
      |             0.928e3;
      |             1.996e3;
      |             1.041e3];  
      | 
      | % Universal gas constant - [J/(mol*K)]   
      | par.R  = 8.314;         
      | 
      | % Specific gas constant [J/kg*K]
      | par.R_j = par.R ./ par.M_j;

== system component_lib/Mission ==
  MN0001_profile : Subsystem  mask{profile=KoblenzTrier.mat, x0=0, N_lookahead=100}
      mask prompts: profile "Road profile:"; x0 "Starting distance [m]:"; N_lookahead "Lookahead horizon [-]:"
      mask init:
      | % find road profiles in folder
      | availableProfiles = dir(fullfile('road_profiles','*.mat'));
      | availableProfiles = {availableProfiles.name};
      | 
      | % update popup_list
      | msk = Simulink.Mask.get(gcb);
      | msk.Parameters(1).TypeOptions = availableProfiles;
      | 
      | % set profile
      | try
      |     load(profile);
      | end
  MN0002_ambient : Subsystem  mask{p_0=1.01e5, T_0=298, RH_0=0.2}
      mask prompts: p_0 "Sea-level pressure [Pa]:"; T_0 "Sea-level temperature [K]:"; RH_0 "Sea-level humidity [-]:"
      mask init:
      | % parameter struct
      | par = struct;
      | 
      | % initial conditions
      | % par.p_0 = eval(get_param(gcb, 'p_0'));
      | % par.T_0 = eval(get_param(gcb, 'T_0'));
      | 
      | par.p_0 = p_0;
      | par.T_0 = T_0;

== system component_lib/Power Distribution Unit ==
  I_load [A] : Inport
  V_bat [V] : Inport  Port=2
  V_fc [V] : Inport  Port=3
  d [-] : Inport  Port=4
  bf [-] : Inport  Port=5
  Add : Sum
  Buck Converter : $bdroot/Electrochemistry/EL0004_buckCCM  R=1e-3  C=1  L=1e-3  V_init=340
  DC Bus : $bdroot/Electrochemistry/EL0006_busDC  R=1e-2  C=1  L=1e-3  V_init=340
  Gain : Gain  Gain=1/R_bf
  Product : Product
  Product1 : Product
  SC0002_signalRead1 : $bdroot/Data & Control/SC0002_signalRead  SigName=burnOffPower
  SC0002_signalRead10 : $bdroot/Data & Control/SC0002_signalRead  SigName=burnOffCurrent
  SC0002_signalRead2 : $bdroot/Data & Control/SC0002_signalRead  SigName=loadCurrent
  SC0002_signalRead3 : $bdroot/Data & Control/SC0002_signalRead  SigName=busVoltage
  Saturation : Saturate  UpperLimit=1  LowerLimit=0  ZeroCross=off
  Sum : Sum  Inputs=++|
  Transfer Fcn : TransferFcn  Denominator=[0.01 1]
  V_bus [V] : Outport
  I_bat [A] : Outport  Port=2
  I_fc [A] : Outport  Port=3
  I_bf [A] : Outport  Port=4
  Q_gen [J/s] : Outport  Port=5
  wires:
  DC Bus/3 -> Buck Converter/2
  V_bat [V]/1 -> DC Bus/1
  d [-]/1 -> Buck Converter/3
  V_fc [V]/1 -> Buck Converter/1
  Buck Converter/2 -> I_fc [A]/1
  DC Bus/1 -> I_bat [A]/1
  DC Bus/2 -> SC0002_signalRead3/1, Product1/2, Product/2, V_bus [V]/1
  Buck Converter/1 -> DC Bus/3
  Buck Converter/3 -> Add/1
  bf [-]/1 -> Saturation/1
  Saturation/1 -> Product/1
  I_load [A]/1 -> SC0002_signalRead2/1, Sum/2
  Sum/1 -> DC Bus/2
  Product/1 -> Gain/1
  Gain/1 -> Transfer Fcn/1
  Transfer Fcn/1 -> I_bf [A]/1, Product1/1, Sum/1, SC0002_signalRead10/1
  Product1/1 -> [Q_bf], SC0002_signalRead1/1
  Add/1 -> Q_gen [J/s]/1
  [Q_bf] -> Add/2

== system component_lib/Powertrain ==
  PT0001_simpleVehicle : Subsystem  mask{m=10e3, r_w=0.5, A_f=10, C_d=0.5, rho_air=1.225, c_r0=0.0060, c_r1=2.3e-7, gain=600, v0=0, x0=0}
      mask prompts: m "Vehicle mass [kg]:"; r_w "Wheel radius [m]:"; A_f "area [m2]:"; C_d "Flow coefficient:"; rho_air "air density [kg/m3]:"; v0 "Initial speed [m/s]:"; x0 "Initial position [m]:"
      mask init:
      | % parameter struct
      | par = struct;
      | 
      | % Get user-defined parameters
      | par.m        = m;
      | par.r_w      = r_w;
      | par.A_f      = A_f;
      | par.C_d      = C_d;
      | par.rho_air  = rho_air;
      | par.c_r0     = c_r0;
      | par.c_r1     = c_r1;
      | par.gain     = gain;
      | par.v0       = v0;
      | par.x0       = x0;
  PT0002_simpleMotor : Subsystem  mask{T_s=0.1}
      mask prompts: T_s "Torque time cont. [s]:"
      mask init:
      | % parameter struct
      | par = struct;
      | 
      | % motor parameters
      | par.e  = 0.86692;
      | par.c1 = 319.3242;
      | par.c2 = -7.3604;
      | par.c3 = 0.060174;
  PT0003_gearBox : Subsystem  mask{fd_ratio=2, gear_ratios=[5 3.8 2.3 1.15], eta_gb=0.98}
      mask prompts: fd_ratio "Final drive ratio [-]:"; gear_ratios "Gear ratios [-]:"; eta_gb "Efficiency [-]:"
      mask init:
      | % parameters
      | par = struct;
      | 
      | par.fd_ratio    = fd_ratio;
      | par.gear_ratios = gear_ratios;
      | par.eta_gb      = eta_gb;
      | par.gears       = 1:length(par.gear_ratios);
  PT0004_electricMachine : Subsystem  mask{T_s=0.1}
      mask prompts: T_s "Torque time cont. [s]:"
      mask init:
      | % parameter struct
      | par = struct;
      | 
      | % motor parameters
      | par.e  = 0.86692;
      | par.c1 = 319.3242;
      | par.c2 = -7.3604;
      | par.c3 = 0.060174;
